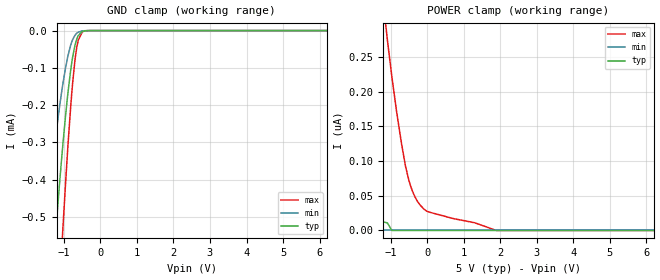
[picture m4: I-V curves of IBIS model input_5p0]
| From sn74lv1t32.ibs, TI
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|   input_5p0 Model
[Model]   input_5p0
Model_type   Input
Vinl = 0.8
Vinh = 2.02
|   typ   min   max
|   (nom PVT)   (fast PVT)   (slow PVT)
C_comp   5.716e-13   5.665e-13   5.768e-13
[Model spec]
|subparameter
Vinl   0.8   0.8   0.8
Vinh   2.02   2.02   2.1
| Where nom  PVT is Nominal Process, 5V, 40C
|   Fast PVT is Strong Process,  5.5V, -40C
|   Slow PVT is Weak Process,   4.5V, 140C
[Voltage Range]   5   4.5   5.5
|Junction Temperature
[Temperature Range]   40   140   -40
[Power Clamp Reference]   5   4.5   5.5
[GND Clamp Reference]   0   0   0
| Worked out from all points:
|   GND clamp passes 1 mA (typ) near -1.55 V on its own axis
[GND Clamp]
|   Voltage   I(typ)   I(min)   I(max)
-5V       -7.607mA   -5.058mA   -9.249mA
-1.553V   -1.008mA   -571.3uA   -1.535mA
-1.47V    -884uA     -493.9uA   -1.367mA
-1.255V   -583.8uA   -308.5uA   -946.7uA
-1.194V   -504.8uA   -260.6uA   -831.9uA
-1.029V   -308.3uA   -144.7uA   -536.1uA
-900mV    -178uA     -73.55uA   -327.2uA
-787mV    -88.65uA   -31.36uA   -172.5uA
-693.5mV  -38.74uA   -12.23uA   -77.66uA
-605.5mV  -13.47uA   -4.237uA   -25.79uA
-319.5mV  -140nA     -88.56nA   -126.5nA
10V       0A         0A         0A
[POWER Clamp]
|   Voltage   I(typ)   I(min)   I(max)
-5V       278.7nA    0A         4.173uA
-4.245V   184.7nA    0A         3.201uA
-3.289V   97.39nA    0A         2.069uA
-2.4V     46.05nA    0A         1.174uA
-1.2V     12.42nA    0A         326.6nA
-1.089V   10.84nA    0A         273.9nA
-968.5mV  0A         0A         221.5nA
-704.5mV  0A         0A         125.3nA
-500mV    0A         0A         71.8nA
5mV       0A         0A         27.46nA
1.891V    0A         0A         0A
10V       0A         0A         0A
